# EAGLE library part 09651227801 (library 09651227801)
D-Sub 9pin male angled 2.54mm pitch, stamped, w/o board locks, M3, PL3 Source: Datasheet
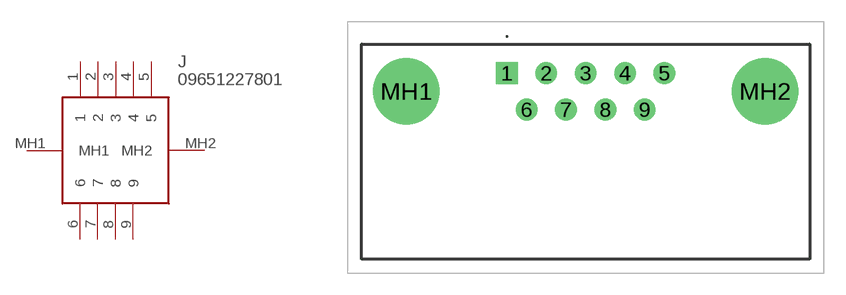
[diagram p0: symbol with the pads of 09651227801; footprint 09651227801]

Designator prefix J

## 09651227801 (Description: D-Sub 9pin male angled 2.54mm pitch, stamped, w/o board locks, M3, PL3; Height: 13.6mm; Manufacturer_Name: HARTING; Manufacturer_Part_Number: 09651227801)  [09651227801]
1  1
2  2
3  3
4  4
5  5
6  6
7  7
8  8
9  9
MH1  MH1
MH2  MH2

## Footprint 09651227801 (pad centres in mm)
09651227801-2
drill 1 pad 1.5 square: 1 0,0
drill 1 pad 1.5: 2 2.74,0; 3 5.48,0; 4 8.22,0; 5 10.96,0; 6 1.37,-2.54; 7 4.11,-2.54; 8 6.85,-2.54; 9 9.59,-2.54
drill 3.1 pad 4.65: MH1 -7.02,-1.27; MH2 17.98,-1.27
